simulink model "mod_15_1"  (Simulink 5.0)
settings: Solver=ode45  StartTime=0.0  StopTime=15.0  FixedStep=1e-6  MaxStep=0.001  RelTol=1e-6

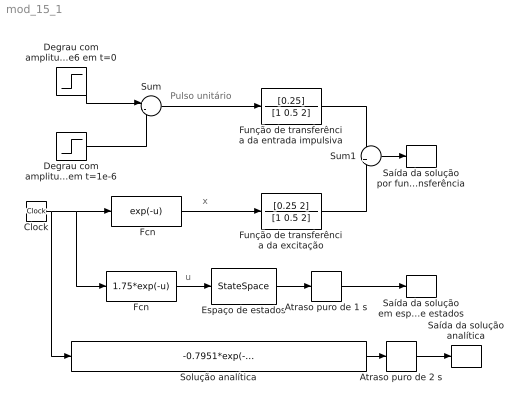
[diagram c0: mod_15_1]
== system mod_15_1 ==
  note: u
  note: Pulso unitário
  note: x
  " Fcn" : Fcn  Expr=exp(-u)
  Atraso puro de 1 s : TransportDelay  BufferSize=16384
  Atraso puro de 2 s : TransportDelay  DelayTime=2  BufferSize=32768
  Clock : Clock
  Degrau com amplitude A=1e6 em t=0 : Step  Time=0  After=1e6  SampleTime=0
  Degrau com amplitude A=1e6 em t=1e-6 : Step  Time=1e-6  After=1e6  SampleTime=0
  Espaço de estados : StateSpace  A=[0 1; -2 -0.5]  B=[0; 1]  C=[1 0]  D=0  X0=[0; 0]
  Fcn : Fcn  Expr=1.75*exp(-u)
  Função de transferência da entrada impulsiva : TransferFcn  Numerator=[0.25]  Denominator=[1 0.5 2]
  Função de transferência da excitação : TransferFcn  Numerator=[0.25 2]  Denominator=[1 0.5 2]
  Saída da solução analítica : ToWorkspace  VariableName=y_an  SampleTime=-1  SaveFormat=Array
  Saída da solução em espaço de estados : ToWorkspace  VariableName=y_ss  SampleTime=-1  SaveFormat=Array
  Saída da solução por funções de transferência : ToWorkspace  VariableName=y_tf  SampleTime=-1  SaveFormat=Array
  Solução analítica : Fcn  Expr=-0.7951*exp(-0.25*u)*cos(1.3919*u+0.4942)+0.7*exp(-u)
  Sum : Sum  Inputs=+-
  Sum1 : Sum  Inputs=-+
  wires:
  Clock/1 -> Solução analítica/1, Fcn/1, " Fcn"/1
  Fcn/1 -> Espaço de estados/1
  Degrau com amplitude A=1e6 em t=0/1 -> Sum/1
  Degrau com amplitude A=1e6 em t=1e-6/1 -> Sum/2
  Sum/1 -> Função de transferência da entrada impulsiva/1
  Sum1/1 -> Saída da solução por funções de transferência/1
  Função de transferência da entrada impulsiva/1 -> Sum1/1
  Função de transferência da excitação/1 -> Sum1/2
  Solução analítica/1 -> Atraso puro de 2 s/1
  Espaço de estados/1 -> Atraso puro de 1 s/1
  Atraso puro de 1 s/1 -> Saída da solução em espaço de estados/1
  Atraso puro de 2 s/1 -> Saída da solução analítica/1
  " Fcn"/1 -> Função de transferência da excitação/1
